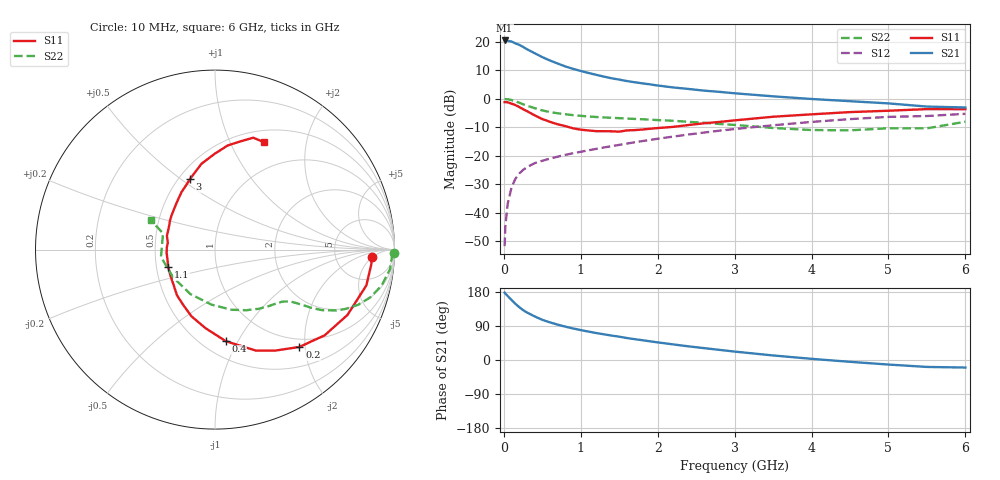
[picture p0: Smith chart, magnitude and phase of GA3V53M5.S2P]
! Infineon Technologies  Discrete & RF Semiconductors
! BF775
! Si NPN RF Bipolar Junction Transistor in SOT23
! VCE = 3.5 V  IC = 3.5 mA
! Common Emitter S-Parameters:  May  1996
# GHz  S  MA  R  50
!  f  S11  S21  S12  S22
! GHz  MAG  ANG  MAG  ANG  MAG  ANG  MAG  ANG
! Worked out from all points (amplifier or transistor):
!   36 points, 10 MHz to 6 GHz, reference 50 ohm
!   highest |S21| = 20.5 dB at 10 MHz (marker M1)
!   |S21| within 3 dB of that: start of sweep to 296.1 MHz
!   unconditionally stable (mu >= 1): 936.9 MHz to 3.529 GHz
!   at 250 MHz: K = 0.40, MSG = 21.6 dB, |S12| = -25.0 dB
!   at 1.4 GHz: K = 1.13, MAG = 9.7 dB, |S12| = -16.6 dB
!   at 6 GHz: K = 0.97, MSG = 1.1 dB, |S12| = -5.3 dB
!   S11 on the Smith chart (normalised r, x): 10 MHz: 13, -5; 200 MHz: 0.84, -1.89; 400 MHz: 0.64, -0.89; 1.1 GHz: 0.58, -0.12; 3 GHz: 0.57, +0.54; 6 GHz: 0.64, +1.35
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0.01  0.8735 -2.7  10.54 177.9  0.0026 91.4  0.9952 -1.2
0.02  0.8747 -5.4  10.37 175.4  0.0059 87.2  0.9863 -2.5
0.05  0.8666 -13.3  10.39 168.9  0.0143 82.7  0.9817 -6.3
0.1  0.8229 -26.3  10.1 158.5  0.0279 76.1  0.95 -12.2
0.15  0.7755 -38.0  9.372 148.2  0.0395 69.6  0.9038 -17.2
0.2  0.7177 -49.1  8.833 139.5  0.0488 65.0  0.8546 -21.1
0.25  0.656 -59.0  8.136 131.7  0.0565 60.7  0.8017 -24.3
0.3  0.6075 -67.9  7.41 125.4  0.0633 58.1  0.7573 -26.6
0.4  0.5136 -83.3  6.305 115.1  0.0741 54.6  0.6849 -29.5
0.5  0.4412 -96.8  5.383 106.0  0.0818 52.7  0.625 -31.2
0.6  0.3943 -109.4  4.693 99.2  0.0892 52.0  0.5845 -32.1
0.7  0.357 -119.4  4.151 93.3  0.0967 51.6  0.557 -32.9
0.9  0.3033 -139.5  3.348 83.2  0.111 51.9  0.5161 -34.3
1.1  0.2782 -159.8  2.838 75.0  0.1248 52.7  0.49 -36.2
1.3  0.2702 -175.4  2.448 67.8  0.1399 53.0  0.4705 -38.2
1.6  0.2786 164.1  2.045 57.9  0.1638 53.1  0.4498 -42.4
2.2  0.3217 135.1  1.581 41.2  0.2171 51.2  0.4116 -53.3
3  0.4183 109.3  1.249 22.2  0.2947 45.0  0.3481 -74.5
3.5  0.4843 98.9  1.104 12.0  0.3432 39.6  0.3072 -93.7
4.5  0.5841 83.1  0.907 -4.8  0.4402 27.1  0.2799 -146.4
5.5  0.659 71.1  0.73 -18.3  0.4986 11.8  0.3032 162.7
6  0.6574 65.6  0.704 -19.9  0.5448 7.6  0.3958 155.1
